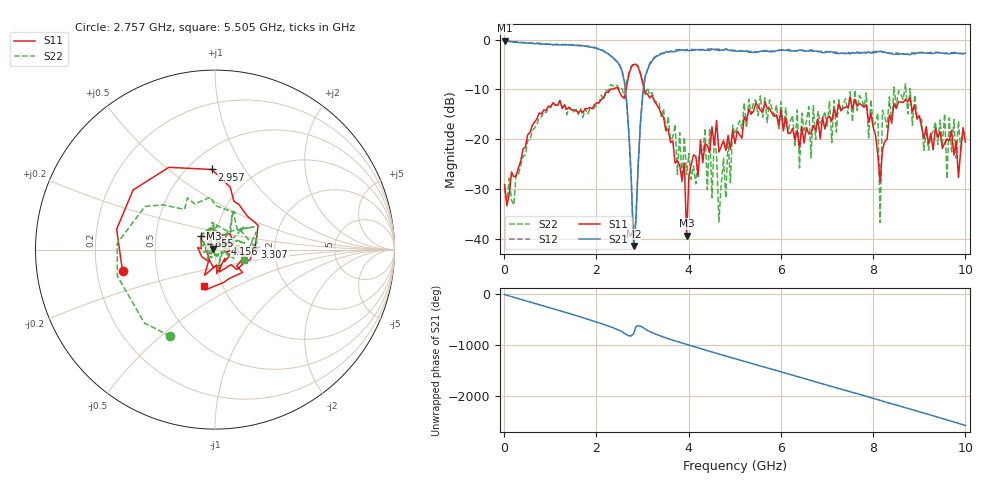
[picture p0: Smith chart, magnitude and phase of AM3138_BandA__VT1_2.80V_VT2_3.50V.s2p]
! Date/Time: Tue, Nov 13, 2018 4:42 PM
! Network Analyzer: Agilent Technologies E8364B Rev: A.07.50.67
! Sweep from 0.010 to 10.000 GHz, 201 Points, Sweep Type: LIN
! Power Supply: 2.801 V, 0.000 A
# Hz S DB R 50
!freq MagS11 AngS11 MagS21 AngS21 MagS12 AngS12 MagS22 AngS22
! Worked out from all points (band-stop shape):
!   201 points, 10 MHz to 10 GHz, reference 50 ohm
!   highest |S21| = -0.23 dB at 10 MHz (marker M1); lowest = -41.5 dB at 2.807 GHz (marker M2)
!   |S21| within 3 dB of the highest: start of sweep to 2.298 GHz; 3.339 GHz to end of sweep
!   lowest |S11| = -39.3 dB at 3.956 GHz (marker M3), VSWR 1.02, Z = 49.1 + j0.569 ohm
!   |S11| at or under -10 dB: start of sweep to 2.303 GHz; 2.475 GHz to 2.643 GHz (167.9 MHz wide, 6.56 % of centre); 3.036 GHz to end of sweep
!   |S22| runs from -36.7 to -4.9 dB; largest |S21 - S12| = 0.028
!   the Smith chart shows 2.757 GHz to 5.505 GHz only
!   S11 on the Smith chart (normalised r, x): 2.757 GHz: 0.31, -0.11; 2.957 GHz: 0.65, +0.72; 3.307 GHz: 1.57, +0.05; 4.156 GHz: 1.12, +0.08; 4.855 GHz: 0.85, +0.13; 5.505 GHz: 0.82, -0.35
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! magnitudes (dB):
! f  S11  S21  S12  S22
! 10 MHz  -29.1  -0.2  -0.2  -29.6
! 1.708 GHz  -14.6  -1.2  -1.2  -15.6
! 2.557 GHz  -11.5  -6.4  -6.3  -9.8
! 2.757 GHz  -5.5  -28.4  -28.2  -5.3
! 2.807 GHz  -5.0  -41.5  -41.5  -4.9
! 2.957 GHz  -7.0  -16.5  -16.5  -6.8
! 3.307 GHz  -13.1  -3.4  -3.3  -12.6
! 3.357 GHz  -13.8  -3.1  -3.0  -12.6
! 3.956 GHz  -39.3  -2.2  -2.0  -27.1
! 4.156 GHz  -23.5  -2.1  -2.0  -29.0
! 4.456 GHz  -22.7  -2.2  -1.9  -17.9
! 4.655 GHz  -22.6  -2.2  -1.9  -36.6
! 4.855 GHz  -19.3  -2.1  -2.0  -20.0
! 5.005 GHz  -20.9  -2.3  -2.1  -19.0
! 5.505 GHz  -13.4  -2.5  -2.4  -15.2
! 6.703 GHz  -17.3  -2.4  -2.2  -13.3
! 7.952 GHz  -14.8  -2.7  -2.5  -12.1
! 8.102 GHz  -23.2  -2.4  -2.4  -14.8
! 8.152 GHz  -28.6  -2.4  -2.3  -36.7
! 8.202 GHz  -22.1  -2.5  -2.4  -14.2
! 8.352 GHz  -15.2  -2.8  -2.8  -11.5
! 10 GHz  -20.6  -2.8  -2.7  -18.9
